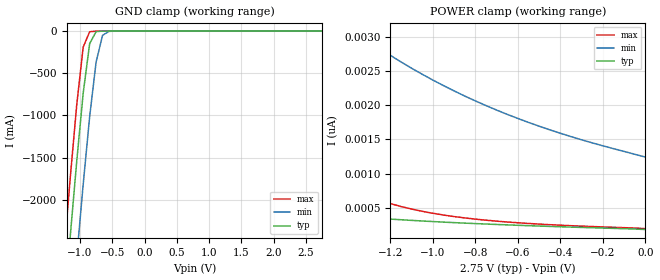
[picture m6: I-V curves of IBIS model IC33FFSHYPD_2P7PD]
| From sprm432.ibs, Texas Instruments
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|   Model IC33FFSHYPD_2P7PD
[Model]   IC33FFSHYPD_2P7PD
Model_type   Input
Polarity   Non-Inverting
Vinl =   0.8250V
Vinh =   1.9250V
C_comp   2.1397pF   2.1767pF   2.7158pF
[Temperature Range]   25.0000   0.1250k   -40.0000
[Voltage Range]   2.7500V   2.5000V   3.0000V
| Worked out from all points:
|   GND clamp passes 1 mA (typ) near -0.66 V on its own axis
[GND_clamp]
| voltage   I(typ)   I(min)   I(max)
-2.75V    -17.91A    -19.01A    -17.27A
-1.25V    -3.342A    -4.502A    -2.646A
-1.15V    -2.424A    -3.58A     -1.732A
-1.05V    -1.541A    -2.68A     -871.7mA
-950mV    -732.7mA   -1.814A    -188.7mA
-850mV    -147.9mA   -1.014A    -7.752mA
-750mV    -6.009mA   -364.9mA   -798.7uA
-650mV    -206.4uA   -49.97mA   -59.18uA
-550mV    -9.486uA   -3.233mA   -2.615uA
2.75V     181.8pA    1.449nA    170.8pA
[POWER_clamp]
| voltage   I(typ)   I(min)   I(max)
-2.75V    1.398nA    9.161nA    24.63nA
-2.4V     922.6pA    6.884nA    9.415nA
-2V       612.2pA    5.001nA    3.237nA
-1.95V    584.8pA    4.808nA    2.846nA
-1.8V     512.9pA    4.278nA    1.955nA
-1.7V     472.6pA    3.961nA    1.538nA
-1.55V    421.6pA    3.534nA    1.095nA
-1.35V    367.1pA    3.045nA    729.7pA
-1.1V     315.3pA    2.541nA    480.7pA
-750mV    261.9pA    1.994nA    318pA
-400mV    222pA      1.589nA    244.9pA
0V        181.8pA    1.241nA    195.1pA
